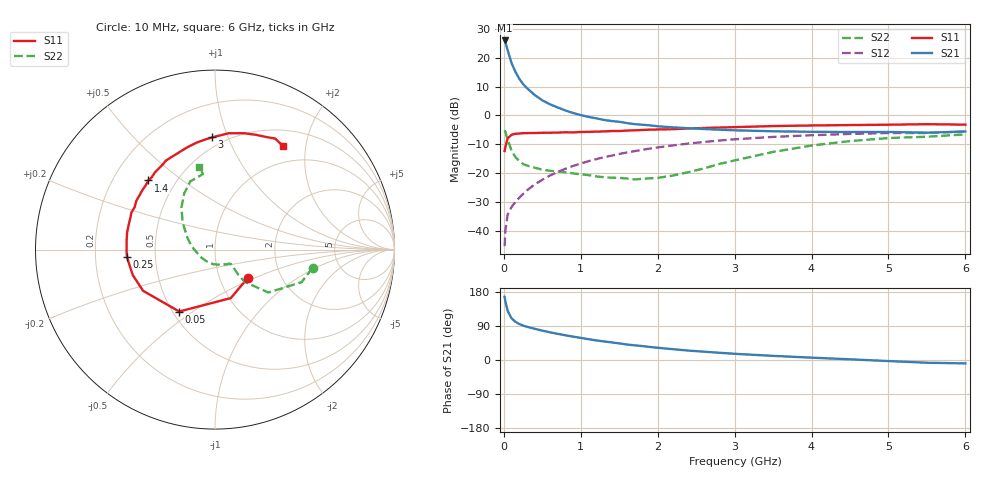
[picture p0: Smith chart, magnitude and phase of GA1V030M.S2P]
! Infineon Technologies  Discrete & RF Semiconductors
! BF775
! Si NPN RF Bipolar Junction Transistor in SOT23
! VCE = 1 V  IC = 30 mA
! Common Emitter S-Parameters:  May  1996
# GHz  S  MA  R  50
!  f  S11  S21  S12  S22
! GHz  MAG  ANG  MAG  ANG  MAG  ANG  MAG  ANG
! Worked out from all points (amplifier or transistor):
!   36 points, 10 MHz to 6 GHz, reference 50 ohm
!   highest |S21| = 26.0 dB at 10 MHz (marker M1)
!   |S21| within 3 dB of that: start of sweep to 45.58 MHz
!   unconditionally stable (mu >= 1): start of sweep to end of sweep
!   at 250 MHz: K = 2.46, MAG = 12.3 dB, |S12| = -27.3 dB
!   at 1.4 GHz: K = 2.27, MAG = -0.3 dB, |S12| = -14.0 dB
!   at 6 GHz: K = 1.20, MAG = -2.7 dB, |S12| = -5.6 dB
!   S11 on the Smith chart (normalised r, x): 10 MHz: 1.35, -0.46; 50 MHz: 0.54, -0.44; 250 MHz: 0.34, -0.03; 1.4 GHz: 0.35, +0.38; 3 GHz: 0.43, +0.88; 6 GHz: 0.72, +1.60
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0.01  0.2414 -41.3  19.91 166.6  0.0054 69.9  0.553 -10.7
0.02  0.2841 -71.9  18.69 154.4  0.0102 66.4  0.5149 -20.7
0.05  0.3984 -120.0  13.42 129.5  0.0191 55.3  0.3813 -38.8
0.1  0.4618 -150.2  8.087 110.2  0.0258 51.7  0.245 -47.4
0.15  0.4795 -162.8  5.707 100.8  0.0316 55.1  0.19 -47.2
0.2  0.4846 -170.0  4.334 95.1  0.0373 58.7  0.1616 -45.4
0.25  0.492 -175.5  3.492 90.9  0.0434 61.3  0.1434 -44.1
0.3  0.4927 -179.0  2.971 87.7  0.0501 63.5  0.1349 -43.2
0.4  0.4949 173.9  2.262 82.4  0.0633 66.0  0.1239 -42.3
0.5  0.4988 169.1  1.826 77.5  0.0765 67.2  0.1144 -43.4
0.6  0.5004 163.8  1.556 73.1  0.0907 67.7  0.1096 -46.1
0.8  0.5095 156.2  1.217 65.3  0.1184 66.5  0.1032 -52.8
0.9  0.5064 152.2  1.101 61.6  0.1327 65.7  0.0987 -56.8
1.1  0.5179 144.3  0.942 55.0  0.1606 63.8  0.0921 -68.3
1.4  0.5349 133.9  0.798 46.5  0.2006 59.7  0.0831 -86.7
1.7  0.551 124.2  0.705 38.7  0.2398 55.4  0.0776 -108.7
2.2  0.577 110.5  0.619 28.5  0.3018 47.4  0.0907 -153.3
3  0.6254 91.5  0.551 16.4  0.3848 34.0  0.1655 157.4
3.5  0.6527 83.3  0.53 10.9  0.4232 26.0  0.2325 140.5
4.5  0.6793 70.2  0.515 1.8  0.4767 11.7  0.3583 118.5
5.5  0.7036 61.5  0.501 -7.2  0.4946 -1.2  0.4263 99.0
6  0.6907 57.0  0.526 -9.0  0.5251 -5.0  0.4688 101.0
